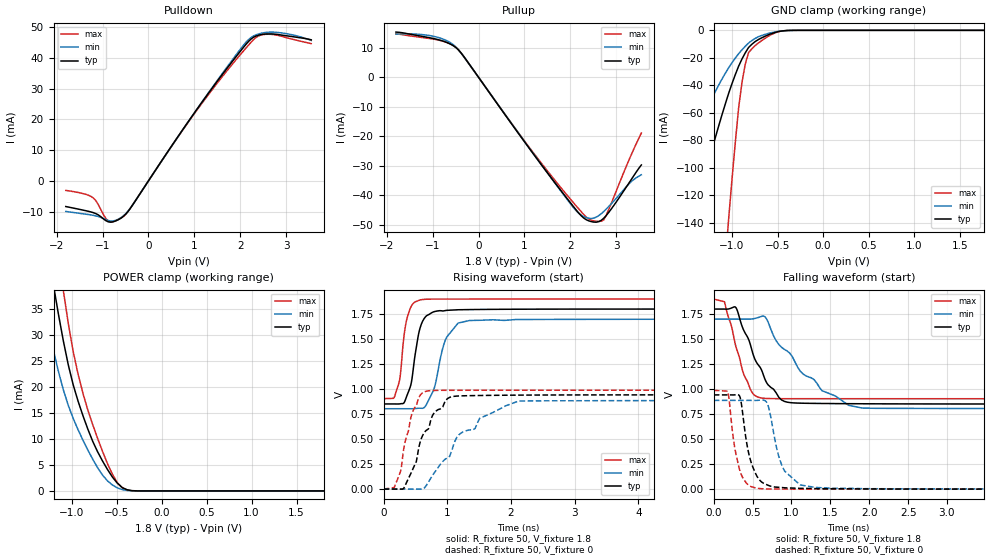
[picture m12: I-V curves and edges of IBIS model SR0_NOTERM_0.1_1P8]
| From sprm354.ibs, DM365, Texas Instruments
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|   Model Cell SR0_NOTERM_0.1_1P8
|SR0_NOTERM_0.1_1P8
[Model]   SR0_NOTERM_0.1_1P8
Model_type   I/O
Polarity   Non-Inverting
Enable   Active-Low
Vinl = 0.8V
Vinh = 2V
Cref =  15.0000pF
Rref =  100.0000M
Vref =  0V
Vmeas =  0.9
C_comp   3.009089p   2.23501p   3.95018p
[Model Spec]
Vinl   0.8V   0.8V   0.8V
Vinh   2V   2V   2V
[Temperature Range]   25   125   -40
[Voltage Range]   1.8   1.7   1.9
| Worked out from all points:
|   slope of the pulldown table from 0 to 0.27 V, typ, clamps not added: 44.1 ohm
|   slope of the pullup table from 0 to 0.27 V, typ, clamps not added: 45.3 ohm
|   GND clamp passes 1 mA (typ) near -0.50 V on its own axis
|   POWER clamp passes 1 mA (typ) near -0.46 V on its own axis
|   rising waveform, R_fixture 50, V_fixture 1.8: 20-80 % time 145ps typ, 212ps min, 111ps max; typ from 0.851 V to 1.8 V
|   rising waveform, R_fixture 50, V_fixture 0: 20-80 % time 334ps typ, 699ps min, 195ps max; typ from 0 V to 0.942 V
|   falling waveform, R_fixture 50, V_fixture 1.8: 20-80 % time 328ps typ, 617ps min, 217ps max; typ from 1.8 V to 0.851 V
|   falling waveform, R_fixture 50, V_fixture 0: 20-80 % time 148ps typ, 178ps min, 120ps max; typ from 0.942 V to 0 V
[POWER_clamp]
|   voltage   I(typ)   I(min)   I(max)
-1.8V     107.1mA    82.35mA    134.1mA
-1.327V   53.28mA    37.61mA    69.48mA
-1.182V   37.78mA    25.71mA    50.1mA
-1.091V   28.94mA    19.51mA    38.64mA
-1.073V   27.41mA    18.51mA    36.54mA
-981.8mV  20.5mA     14.01mA    26.92mA
-872.7mV  14.5mA     9.783mA    18.82mA
-709.1mV  7.513mA    4.449mA    10.09mA
-545.5mV  2.674mA    1.139mA    3.211mA
-436.4mV  654.9uA    255.5uA    594.1uA
-327.3mV  54.9uA     31.45uA    28.9uA
1.8V      5.504nA    121.3nA    1.604nA
[Pulldown]
|   voltage   I(typ)   I(min)   I(max)
-1.8V     -8.351mA   -9.956mA   -3.097mA
-1.2V     -10.35mA   -11.23mA   -5.575mA
-872.7mV  -13.35mA   -12.93mA   -13.07mA
-763.6mV  -13.31mA   -13.05mA   -13.22mA
-600mV    -12.16mA   -11.98mA   -12.14mA
-381.8mV  -8.669mA   -8.593mA   -8.643mA
1.145V    25.19mA    25.27mA    24.87mA
2.182V    45.44mA    46.03mA    44.25mA
2.345V    47.19mA    47.58mA    46.72mA
2.564V    47.83mA    48.35mA    47.74mA
3V        47.27mA    47.96mA    46.66mA
3.545V    45.94mA    45.74mA    44.7mA
[Pullup]
|   voltage   I(typ)   I(min)   I(max)
-1.8V     15.34mA    14.64mA    14.75mA
-981.8mV  13.15mA    13.91mA    12.94mA
-709.1mV  11.92mA    12.55mA    11.92mA
-490.9mV  10.05mA    10.24mA    10.12mA
1.145V    -24.96mA   -24.87mA   -24.59mA
2.018V    -42.87mA   -43.22mA   -41.64mA
2.236V    -46.95mA   -46.75mA   -45.58mA
2.455V    -48.93mA   -47.86mA   -48.45mA
2.618V    -48.93mA   -46.89mA   -48.85mA
2.727V    -47.76mA   -45.48mA   -48.34mA
3.273V    -35.91mA   -36.16mA   -28.15mA
3.545V    -29.71mA   -33.05mA   -18.91mA
[GND_clamp]
|   voltage   I(typ)   I(min)   I(max)
-1.8V     -229.3mA   -132mA     -818.5mA
-1.436V   -139.1mA   -79.12mA   -490.7mA
-1.073V   -53.39mA   -31.17mA   -167.2mA
-1.036V   -45.75mA   -27.16mA   -136.8mA
-927.3mV  -26.08mA   -17mA      -56.49mA
-890.9mV  -20.9mA    -14.21mA   -38.02mA
-854.5mV  -16.38mA   -11.64mA   -24.6mA
-818.2mV  -12.5mA    -9.275mA   -16.24mA
-709.1mV  -6.663mA   -4.641mA   -9.157mA
-527.3mV  -1.534mA   -1.158mA   -1.867mA
-381.8mV  -101.4uA   -119.7uA   -85.8uA
1.764V    4.755nA    203.2nA    1.222nA
[Ramp]
| variable   typ   min   max
dV/dt_f  0.5831644/0.3322235n  0.5557921/0.6253163n  0.6085253/0.2208185n
dV/dt_r  0.5657631/0.3333447n  0.5323474/0.6989629n   0.593735/0.1939523n
R_load = 50
[Rising Waveform]
R_fixture = 50
V_fixture = 1.8
V_fixture_min = 1.7
V_fixture_max = 1.9
|   time   V(typ)   V(min)   V(max)
0s        851mV      803.4mV    903.9mV
156ps     851mV      803.4mV    907.5mV
233.6ps   850.9mV    803.4mV    1.048V
328.8ps   872.9mV    803.4mV    1.576V
436ps     1.069V     803.1mV    1.831V
570.4ps   1.608V     808.7mV    1.891V
779.2ps   1.771V     984.9mV    1.9V
967.2ps   1.785V     1.487V     1.9V
1.17ns    1.793V     1.66V      1.9V
5.34ns    1.8V       1.698V     1.9V
[Rising Waveform]
R_fixture = 50
V_fixture = 0
V_fixture_min = 0
V_fixture_max = 0
|   time   V(typ)   V(min)   V(max)
0s        84.48nV    277.7nV    33.22nV
165.6ps   3.928uV    340.3nV    14.93mV
265.6ps   -796.4uV   -405.1nV   178.8mV
315.2ps   7.921mV    478.5nV    402.1mV
452.8ps   191.7mV    -796.4uV   769.6mV
671.2ps   588.3mV    37.28mV    978.6mV
1.036ns   916.8mV    327.3mV    987.6mV
1.218ns   931.9mV    561.5mV    987.9mV
2.119ns   939.3mV    880.4mV    988.3mV
6.39ns    942mV      885.5mV    988.3mV
[Falling Waveform]
R_fixture = 50
V_fixture = 1.8
V_fixture_min = 1.7
V_fixture_max = 1.9
|   time   V(typ)   V(min)   V(max)
0s        1.8V       1.7V       1.9V
137.6ps   1.8V       1.7V       1.873V
286.4ps   1.813V     1.7V       1.42V
469.6ps   1.448V     1.699V     1V
598.4ps   1.215V     1.723V     913.6mV
670.4ps   1.078V     1.712V     906.9mV
907.2ps   877.9mV    1.398V     904.4mV
1.393ns   856.4mV    984.3mV    904.2mV
1.737ns   854.3mV    837.7mV    904mV
5.518ns   851mV      805.1mV    903.9mV
[Falling Waveform]
R_fixture = 50
V_fixture = 0
V_fixture_min = 0
V_fixture_max = 0
|   time   V(typ)   V(min)   V(max)
0s        942mV      887.2mV    988.3mV
178.4ps   942mV      887.2mV    979.3mV
260.8ps   941.9mV    887.2mV    458.8mV
330.4ps   933.1mV    887.2mV    200.8mV
444ps     378mV      887.2mV    42.37mV
539.2ps   154.3mV    886.9mV    12.39mV
676ps     46.71mV    873.8mV    2.816mV
872.8ps   16.74mV    245.1mV    981.9uV
1.11ns    8.206mV    42.99mV    376.6uV
5.66ns    83.77uV    1.701mV    30.92nV
